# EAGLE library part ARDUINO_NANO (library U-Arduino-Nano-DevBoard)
Arduino Nano, Through Hole and SMT.
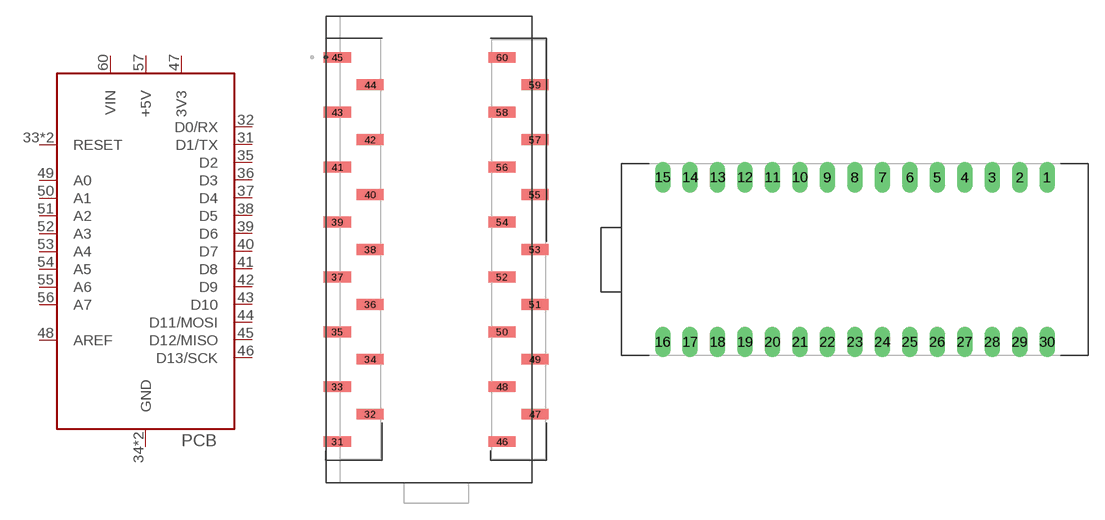
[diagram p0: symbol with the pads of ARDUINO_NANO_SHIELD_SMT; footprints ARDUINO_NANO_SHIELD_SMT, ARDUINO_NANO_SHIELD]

Designator prefix PCB

## ARDUINO_NANOSMT (AVAILABILITY: Unavailable; DESCRIPTION: Dev.kit: Arduino; UART; ICSP, USB B mini, pin strips; MF: Arduino; MP: ARDUINO NANO; PACKAGE: None; PRICE: None)  [ARDUINO_NANO_SHIELD_SMT]
31  D1/TX
32  D0/RX
33  RESET  in
34  GND  pwr
35  D2
36  D3
37  D4
38  D5
39  D6
40  D7
41  D8
42  D9
43  D10
44  D11/MOSI
45  D12/MISO
46  D13/SCK
47  3V3  pwr
48  AREF  pwr
49  A0  in
50  A1  in
51  A2  in
52  A3  in
53  A4  in
54  A5  in
55  A6  in
56  A7  in
57  +5V  pwr
58  RESET  in
59  GND  pwr
60  VIN  pwr

## ARDUINO_NANO  [ARDUINO_NANO_SHIELD]
1  D1/TX
2  D0/RX
3  RESET  in
4  GND  pwr
5  D2
6  D3
7  D4
8  D5
9  D6
10  D7
11  D8
12  D9
13  D10
14  D11/MOSI
15  D12/MISO
16  D13/SCK
17  3V3  pwr
18  AREF  pwr
19  A0  in
20  A1  in
21  A2  in
22  A3  in
23  A4  in
24  A5  in
25  A6  in
26  A7  in
27  +5V  pwr
28  RESET  in
29  GND  pwr
30  VIN  pwr

## Footprint ARDUINO_NANO_SHIELD_SMT (pad centres in mm)
smd 2.5 x 1: 31 -9.14,-17.78; 32 -6.1,-15.24; 33 -9.14,-12.7; 34 -6.1,-10.16; 35 -9.14,-7.62; 36 -6.1,-5.08; 37 -9.14,-2.54; 38 -6.1,0; 39 -9.14,2.54; 40 -6.1,5.08; 41 -9.14,7.62; 42 -6.1,10.16; 43 -9.14,12.7; 44 -6.1,15.24; 45 -9.14,17.78; 46 6.1,-17.78; 47 9.14,-15.24; 48 6.1,-12.7; 49 9.14,-10.16; 50 6.1,-7.62; 51 9.14,-5.08; 52 6.1,-2.54; 53 9.14,0; 54 6.1,2.54; 55 9.14,5.08; 56 6.1,7.62; 57 9.14,10.16; 58 6.1,12.7; 59 9.14,15.24; 60 6.1,17.78

## Footprint ARDUINO_NANO_SHIELD (pad centres in mm)
drill 0.914 long: 1 19.05,7.62; 2 16.51,7.62; 3 13.97,7.62; 4 11.43,7.62; 5 8.89,7.62; 6 6.35,7.62; 7 3.81,7.62; 8 1.27,7.62; 9 -1.27,7.62; 10 -3.81,7.62; 11 -6.35,7.62; 12 -8.89,7.62; 13 -11.43,7.62; 14 -13.97,7.62; 15 -16.51,7.62; 16 -16.51,-7.62; 17 -13.97,-7.62; 18 -11.43,-7.62; 19 -8.89,-7.62; 20 -6.35,-7.62; 21 -3.81,-7.62; 22 -1.27,-7.62; 23 1.27,-7.62; 24 3.81,-7.62; 25 6.35,-7.62; 26 8.89,-7.62; 27 11.43,-7.62; 28 13.97,-7.62; 29 16.51,-7.62; 30 19.05,-7.62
